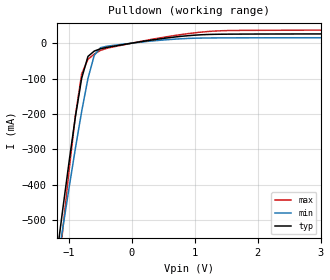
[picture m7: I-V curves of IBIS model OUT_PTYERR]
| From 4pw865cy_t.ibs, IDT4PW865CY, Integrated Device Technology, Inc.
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|   Model OUT_PTYERR
[Model]   OUT_PTYERR
Model_type   Open_sink
Polarity   Inverting
C_comp   6.50000pF   8.10000pF   5.40000pF
[Temperature Range]   25.00000   0.11000k   0.000
[Voltage Range]   1.80000V   1.70000V   1.90000V
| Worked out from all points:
|   slope of the pulldown table from 0 to 0.27 V, typ, clamps not added: 35.5 ohm
[Pulldown]
| voltage   I(typ)   I(min)   I(max)
-1.8V     -1.472A    -1.355A    -1.781A
-1.2V     -606.1mA   -638.3mA   -697.7mA
-1.1V     -468.1mA   -522.1mA   -525.5mA
-1V       -334.5mA   -408.1mA   -359mA
-900mV    -208.2mA   -297.4mA   -204.7mA
-800mV    -98.98mA   -192.6mA   -86.78mA
-700mV    -37.53mA   -99.73mA   -45.51mA
-600mV    -22.44mA   -34.39mA   -30.96mA
-500mV    -15.88mA   -12.82mA   -20.56mA
400mV     10.95mA    7.405mA    13.4mA
1.2V      24.39mA    14.57mA    32.73mA
3.6V      26.18mA    15.42mA    36.84mA
[Ramp]
| variable   typ   min   max
dV/dt_r   0.59166/0.40463n   0.41880/0.62083n   0.69480/0.35195n
dV/dt_f   0.59202/0.64654n   0.41220/1.11029n   0.69540/0.41713n
R_load = 50.00000
| End [Model] OUT_PTYERR
